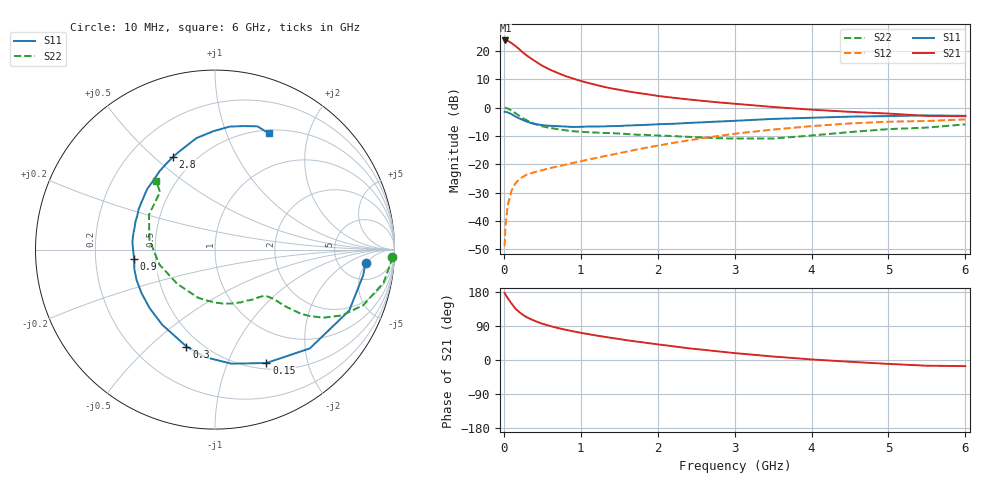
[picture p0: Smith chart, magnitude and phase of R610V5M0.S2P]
! SIEMENS Small Signal Semiconductors
! BFR193
! Si NPN RF Bipolar Junction Transistor in SOT23
! VCE = 10 V  IC = 5 mA
! Common Emitter S-Parameters:  May  1996
# GHz  S  MA  R  50
!  f  S11  S21  S12  S22
! GHz  MAG  ANG  MAG  ANG  MAG  ANG  MAG  ANG
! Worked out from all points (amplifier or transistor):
!   36 points, 10 MHz to 6 GHz, reference 50 ohm
!   highest |S21| = 23.6 dB at 20 MHz (marker M1)
!   |S21| within 3 dB of that: start of sweep to 197.8 MHz
!   unconditionally stable (mu >= 1): 916.9 MHz to 2.044 GHz
!   at 250 MHz: K = 0.42, MSG = 21.9 dB, |S12| = -24.4 dB
!   at 1.4 GHz: K = 1.07, MAG = 10.1 dB, |S12| = -16.7 dB
!   at 6 GHz: K = 0.95, MSG = 0.6 dB, |S12| = -4.2 dB
!   S11 on the Smith chart (normalised r, x): 10 MHz: 9, -5; 150 MHz: 0.57, -1.39; 300 MHz: 0.42, -0.66; 900 MHz: 0.38, -0.05; 2.8 GHz: 0.38, +0.58; 6 GHz: 0.54, +1.42
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0.01  0.8423 -4.9  15.17 176.8  0.0036 83.5  0.9875 -2.3
0.02  0.838 -9.8  15.19 173.0  0.0078 81.4  0.9813 -4.5
0.05  0.8214 -24.4  15.02 163.4  0.0187 77.5  0.9572 -11.1
0.1  0.7631 -46.2  13.65 149.0  0.0343 68.1  0.8828 -20.5
0.15  0.6937 -65.6  12.14 135.9  0.046 59.9  0.7967 -27.4
0.2  0.6425 -81.7  10.7 126.4  0.0546 54.7  0.7137 -32.1
0.25  0.6016 -95.4  9.265 118.8  0.0603 51.0  0.6464 -35.0
0.3  0.5628 -106.4  8.201 112.5  0.0658 49.1  0.5956 -36.8
0.4  0.5117 -125.1  6.637 103.3  0.0725 47.9  0.5154 -38.6
0.5  0.489 -138.1  5.446 95.8  0.0787 47.7  0.4644 -39.5
0.6  0.4759 -149.3  4.645 89.8  0.0855 48.7  0.437 -39.9
0.7  0.4689 -158.7  4.062 84.5  0.0915 50.0  0.4151 -40.6
0.9  0.4535 -173.2  3.237 75.7  0.1057 53.4  0.3819 -42.5
1.1  0.4623 174.6  2.702 68.2  0.121 55.8  0.3667 -45.6
1.3  0.4645 164.7  2.317 61.5  0.1384 57.5  0.3562 -49.0
1.6  0.4814 152.0  1.936 52.1  0.1671 58.8  0.3411 -56.0
2.2  0.5162 131.7  1.487 36.2  0.2375 57.5  0.3136 -73.8
2.8  0.5668 114.5  1.228 22.5  0.3167 51.8  0.2871 -99.0
3.5  0.6297 99.5  1.022 9.2  0.4084 41.7  0.2842 -137.6
4.5  0.6902 83.2  0.839 -4.7  0.5238 25.4  0.3693 171.5
5.5  0.7264 71.0  0.711 -15.1  0.5783 8.2  0.4428 133.8
6  0.7139 65.3  0.703 -16.2  0.6171 3.2  0.5041 130.4
